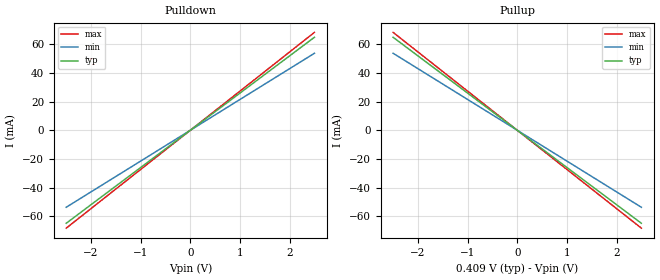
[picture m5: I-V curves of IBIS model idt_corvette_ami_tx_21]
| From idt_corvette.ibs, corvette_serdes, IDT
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|   model   idt_corvette_ami_tx_21
[Model] idt_corvette_ami_tx_21
Model_type Output
C_comp 400f 400f 400f
Cref = 0
[Model Spec]
Vmeas 0. 0. 0.
Vref 0. 0. 0.
[Temperature Range]  25 100 0
[Voltage Range] .409 .41 .354
[Algorithmic Model]
Executable Windows_VisualStudio5_32 idt_corvette_tx.dll   idt_corvette_tx.ami
Executable Windows_ver_64   idt_corvette_tx_64.dll   idt_corvette_tx.ami
Executable Linux_gcc4.1.2_32   idt_corvette_tx.linux.so   idt_corvette_tx.ami
Executable Linux_gcc3.2.3_64   idt_corvette_tx_64.linux.so idt_corvette_tx.ami
[End Algorithmic Model]
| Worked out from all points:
|   slope of the pulldown table from 0 to 0.061 V, typ, clamps not added: 38.5 ohm
|   slope of the pullup table from 0 to 0.061 V, typ, clamps not added: 38.5 ohm
[Pulldown]
-2.5V     -64.94mA   -53.76mA   -68.35mA
0V        0A         0A         0A
2.5V      64.94mA    53.76mA    68.35mA
[Pullup]
-2.5V     64.94mA    53.76mA    68.35mA
0V        0A         0A         0A
2.5V      -64.94mA   -53.76mA   -68.35mA
[Ramp]
dV/dt_r .139/21.56p .128/26.04p .123/20.483p
dV/dt_f .139/21.56p .128/26.04p .123/20.483p
